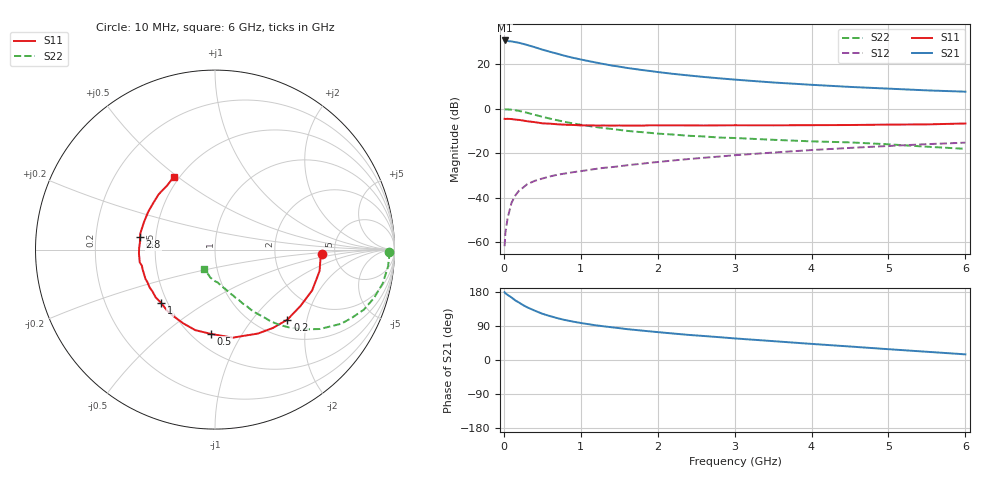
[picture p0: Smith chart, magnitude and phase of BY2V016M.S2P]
! SIEMENS Small Signal Semiconductors
! BFY420
! Si NPN RF SIEGET Grounded Emitter Transistor in MICRO-X
! VCE = 2 V  IC = 16 mA
! Common Emitter S-Parameters:  October  1996
# GHz  S  MA  R  50
!  f  S11  S21  S12  S22
! GHz  MAG  ANG  MAG  ANG  MAG  ANG  MAG  ANG
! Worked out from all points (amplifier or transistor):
!   36 points, 10 MHz to 6 GHz, reference 50 ohm
!   highest |S21| = 30.8 dB at 10 MHz (marker M1)
!   |S21| within 3 dB of that: start of sweep to 398.2 MHz
!   unconditionally stable (mu >= 1): 2.112 GHz to end of sweep
!   at 250 MHz: K = 0.27, MSG = 32.4 dB, |S12| = -35.5 dB
!   at 1.4 GHz: K = 0.87, MSG = 22.9 dB, |S12| = -26.3 dB
!   at 6 GHz: K = 1.08, MAG = 9.7 dB, |S12| = -15.3 dB
!   S11 on the Smith chart (normalised r, x): 10 MHz: 3.91, -0.33; 200 MHz: 1.35, -1.53; 500 MHz: 0.62, -0.74; 1 GHz: 0.46, -0.34; 2.8 GHz: 0.41, +0.07; 6 GHz: 0.47, +0.48
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0.01  0.5949 -2.6  34.73 178.8  0.0008 103.8  0.9676 -0.7
0.02  0.5898 -4.9  34.6 176.1  0.0016 90.9  0.9719 -1.9
0.05  0.5948 -11.5  33.66 171.7  0.0035 86.8  0.9688 -5.5
0.1  0.5871 -22.8  33.01 165.1  0.0076 82.0  0.9534 -11.4
0.15  0.5704 -33.5  31.83 157.1  0.0112 76.1  0.9261 -16.9
0.2  0.5612 -44.1  30.68 151.3  0.0144 73.0  0.8949 -21.9
0.25  0.5429 -53.5  29.12 144.9  0.0167 67.5  0.8528 -26.4
0.3  0.5256 -62.8  27.56 139.4  0.0198 66.7  0.8158 -30.4
0.4  0.5005 -78.6  24.53 130.4  0.0237 62.2  0.7334 -37.1
0.5  0.4705 -92.6  21.58 122.1  0.0268 59.1  0.661 -42.3
0.6  0.4621 -103.7  19.3 115.8  0.0299 57.2  0.6006 -46.3
0.7  0.4475 -113.2  17.33 110.2  0.0327 55.8  0.5496 -49.6
0.8  0.4372 -122.1  15.55 105.3  0.0349 54.1  0.5048 -52.2
1  0.4225 -134.9  12.94 97.7  0.0393 54.5  0.4378 -55.9
1.1  0.4243 -141.2  11.93 94.5  0.0417 54.4  0.4111 -57.8
1.6  0.418 -161.4  8.349 81.5  0.0533 54.0  0.3186 -64.1
2.2  0.4242 -177.2  6.135 69.9  0.0684 52.8  0.2626 -70.2
2.8  0.4234 170.6  4.867 60.2  0.0839 50.2  0.225 -75.5
3.5  0.4244 158.6  3.921 49.8  0.1032 46.2  0.2001 -81.4
4.5  0.4309 143.0  3.115 35.6  0.1314 38.6  0.1749 -90.6
5.5  0.4454 126.8  2.601 21.7  0.1595 29.7  0.1398 -106.9
6  0.4663 119.5  2.432 14.9  0.1726 24.9  0.1251 -118.8
